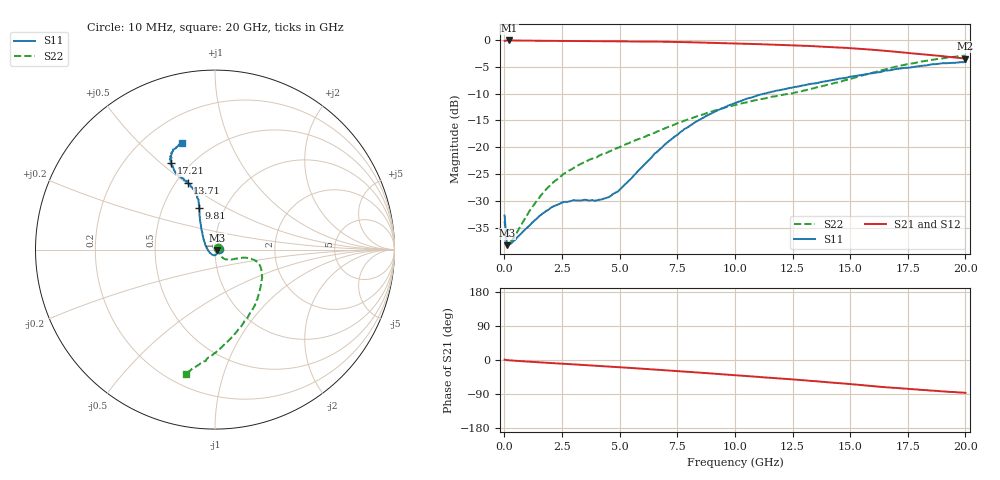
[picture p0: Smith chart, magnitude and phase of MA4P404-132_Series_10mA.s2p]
! AWR Design Environment (9226) Thu Aug 19 02:30:18 2021
! Document = '10mA'
! nPorts: 2, nXvals: 201
# GHz S DB R 50
!Freq DBS11 AngS11 DBS21 AngS21 DBS12 AngS12 DBS22 AngS22
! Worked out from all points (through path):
!   201 points, 10 MHz to 20 GHz, reference 50 ohm
!   highest |S21| = -0.16 dB at 210 MHz (marker M1); lowest = -3.5 dB at 20 GHz (marker M2)
!   group delay of S21, straight-line fit = 12.2 ps
!   lowest |S11| = -38.2 dB at 110 MHz (marker M3), VSWR 1.02, Z = 51.2 - j0.141 ohm
!   |S11| at or under -10 dB: start of sweep to 11.3 GHz
!   |S22| runs from -38.3 to -3.0 dB; largest |S21 - S12| = 0.034
!   S11 on the Smith chart (normalised r, x): 10 MHz: 1.05, +0.01; 9.81 GHz: 0.76, +0.37; 13.71 GHz: 0.57, +0.51; 17.21 GHz: 0.40, +0.54; 20 GHz: 0.35, +0.68
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0.01  -32.63 7.5  -0.23 1.1  -0.22 0.8  -33.66 23.6
0.11  -38.19 -6.4  -0.16 -0.4  -0.15 -0.5  -38.32 -6.4
0.21  -38.03 -9.5  -0.16 -0.9  -0.15 -0.9  -37.82 -9.7
1.21  -33.93 -49.4  -0.20 -4.9  -0.18 -4.8  -31.05 -38.7
1.81  -31.80 -66.7  -0.23 -7.2  -0.21 -6.9  -27.79 -44.2
2.51  -30.22 -85.5  -0.25 -9.8  -0.24 -9.4  -25.10 -47.3
3.41  -29.76 -110.8  -0.27 -13.1  -0.26 -12.6  -22.86 -44.8
4.21  -29.67 -143.5  -0.29 -16.0  -0.28 -15.5  -21.32 -39.7
4.91  -28.21 -175.0  -0.31 -18.8  -0.30 -18.1  -20.08 -34.3
6.71  -20.50 134.1  -0.38 -26.0  -0.37 -25.1  -16.92 -19.5
7.81  -16.58 121.6  -0.47 -30.6  -0.46 -29.6  -15.01 -14.8
8.81  -14.05 115.2  -0.57 -34.8  -0.56 -33.6  -13.59 -14.1
9.81  -12.09 111.0  -0.68 -39.2  -0.67 -37.7  -12.35 -16.0
10.01  -11.77 109.7  -0.71 -40.2  -0.69 -38.6  -12.14 -16.1
11.71  -9.57 108.9  -0.95 -47.5  -0.88 -45.9  -10.55 -27.9
13.41  -8.15 111.8  -1.22 -55.4  -1.13 -53.8  -9.02 -47.1
13.71  -7.89 112.2  -1.29 -57.1  -1.19 -55.2  -8.73 -50.9
14.81  -7.10 115.0  -1.53 -62.5  -1.42 -60.8  -7.50 -64.7
16.71  -5.70 117.2  -2.15 -72.7  -2.03 -71.0  -5.31 -85.8
17.21  -5.33 116.7  -2.35 -74.9  -2.24 -73.6  -4.80 -89.8
18.71  -4.55 114.2  -2.97 -81.2  -2.95 -80.8  -3.62 -99.1
20  -4.15 107.3  -3.51 -86.7  -3.61 -85.9  -2.96 -103.0
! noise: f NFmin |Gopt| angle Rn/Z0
0.01  0  1  0  2e-20
2.21  0  1  0  2e-20
4.41  0  1  0  2e-20
6.61  0  1  0  2e-20
8.81  0  1  0  2e-20
11.11  0  1  0  2e-20
13.31  0  1  0  2e-20
15.51  0  1  0  2e-20
17.71  0  1  0  2e-20
20  0  1  0  2e-20
